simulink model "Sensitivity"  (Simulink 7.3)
settings: Solver=ode5  StartTime=0.0  StopTime=100  FixedStep=0.04  RelTol=1e-3
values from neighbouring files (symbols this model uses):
  Ts = 0.04    [run.m]    (also in z2s_transf.m)
undefined symbols (not defined in the file or in its folder): Alfc, Apfc, Azpl, Blfc, Bpfc, Bzpl, Clfc, Cpfc, Czpl, Dlfc, Dpfc, Dzpl, TVC

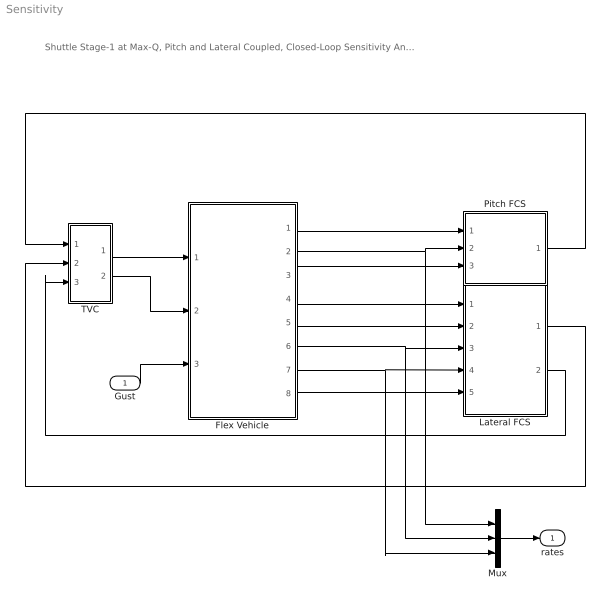
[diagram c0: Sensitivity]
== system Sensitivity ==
  note: Shuttle Stage-1 at Max-Q, Pitch and Lateral Coupled, Closed-Loop Sensitivity Analysis Model
  Gust : Inport  OutDataType=sfix(16)  OutScaling=2^0
  Flex Vehicle : Subsystem
  Lateral FCS : Subsystem
  Mux : Mux  Inputs=3
  Pitch FCS : Subsystem
  TVC : Subsystem
  rates : Outport  OutDataType=sfix(16)  OutScaling=2^0
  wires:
  Pitch FCS/1(DQ_TVC) -> TVC/1(ptch)
  Lateral FCS/1(DP_TVC) -> TVC/2(roll)
  Lateral FCS/2(DR_TVC) -> TVC/3(yaw)
  TVC/2(dz) -> Flex Vehicle/2(dzc)
  TVC/1(dy) -> Flex Vehicle/1(dyc)
  Flex Vehicle/2(q-flx) -> Mux/1, Pitch FCS/2(q)
  Flex Vehicle/3(Nz) -> Pitch FCS/3(Nz)
  Flex Vehicle/4(phi) -> Lateral FCS/1(phi-er)
  Flex Vehicle/5(psi) -> Lateral FCS/2(psi-er)
  Flex Vehicle/6(p-flx) -> Mux/2, Lateral FCS/3(p)
  Flex Vehicle/7(r-flx) -> Mux/3, Lateral FCS/4(r)
  Flex Vehicle/8(Ny) -> Lateral FCS/5(Ny)
  Gust/1 -> Flex Vehicle/3(WG)
  Mux/1 -> rates/1
  Flex Vehicle/1(theta) -> Pitch FCS/1(theta)

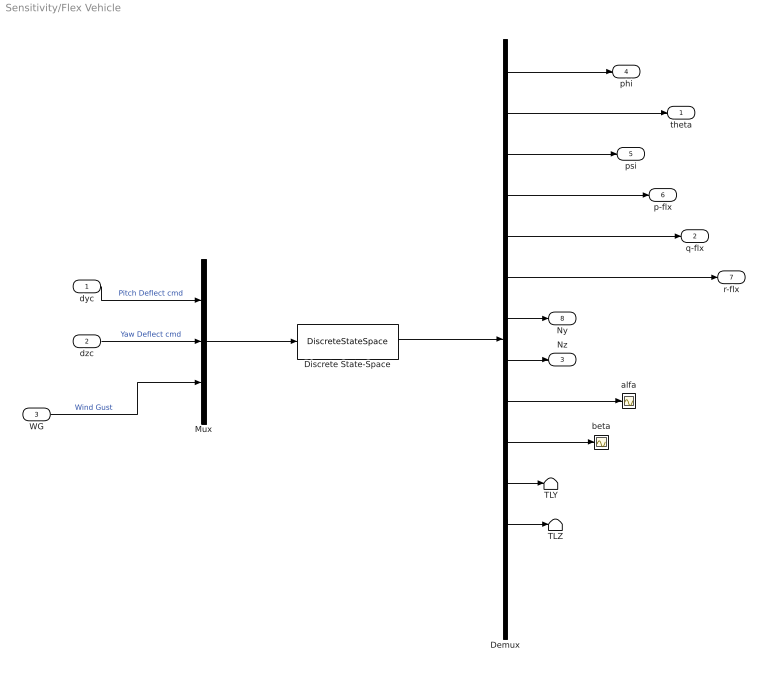
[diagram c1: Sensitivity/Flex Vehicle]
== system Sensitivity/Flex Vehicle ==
  dyc : Inport  PortDimensions=5  OutDataType=sfix(16)  OutScaling=2^0
  dzc : Inport  Port=2  PortDimensions=5  OutDataType=sfix(16)  OutScaling=2^0
  WG : Inport  Port=3  OutDataType=sfix(16)  OutScaling=2^0
  Demux : Demux  Outputs=[1,1,1,1,1,1,1,1,1,1, 5,5,5,5]
  Discrete State-Space : DiscreteStateSpace  A=Azpl  B=Bzpl  C=Czpl  D=Dzpl  SampleTime=Ts
  Mux : Mux  Inputs="[5  5  1]"
  TLY : Terminator
  TLZ : Terminator
  alfa : Scope
  beta : Scope
  theta : Outport  OutDataType=sfix(16)  OutScaling=2^0
  q-flx : Outport  Port=2  OutDataType=sfix(16)  OutScaling=2^0
  Nz : Outport  Port=3  OutDataType=sfix(16)  OutScaling=2^0
  phi : Outport  Port=4  OutDataType=sfix(16)  OutScaling=2^0
  psi : Outport  Port=5  OutDataType=sfix(16)  OutScaling=2^0
  p-flx : Outport  Port=6  OutDataType=sfix(16)  OutScaling=2^0
  r-flx : Outport  Port=7  OutDataType=sfix(16)  OutScaling=2^0
  Ny : Outport  Port=8  OutDataType=sfix(16)  OutScaling=2^0
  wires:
  dyc/1 -> Mux/1  "Pitch Deflect cmd"
  dzc/1 -> Mux/2  "Yaw Deflect cmd"
  WG/1 -> Mux/3  "Wind Gust"
  Mux/1 -> Discrete State-Space/1
  Discrete State-Space/1 -> Demux/1
  Demux/1 -> phi/1
  Demux/2 -> theta/1
  Demux/3 -> psi/1
  Demux/4 -> p-flx/1
  Demux/5 -> q-flx/1
  Demux/6 -> r-flx/1
  Demux/7 -> Ny/1
  Demux/8 -> Nz/1
  Demux/9 -> alfa/1
  Demux/10 -> beta/1
  Demux/11 -> TLY/1
  Demux/12 -> TLZ/1

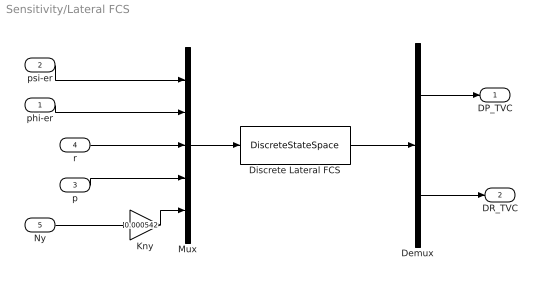
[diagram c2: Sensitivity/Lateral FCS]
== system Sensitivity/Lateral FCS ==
  phi-er : Inport  OutDataType=sfix(16)  OutScaling=2^0
  psi-er : Inport  Port=2  OutDataType=sfix(16)  OutScaling=2^0
  p : Inport  Port=3  OutDataType=sfix(16)  OutScaling=2^0
  r : Inport  Port=4  OutDataType=sfix(16)  OutScaling=2^0
  Ny : Inport  Port=5  OutDataType=sfix(16)  OutScaling=2^0
  Demux : Demux  Outputs=2
  Discrete Lateral FCS : DiscreteStateSpace  A=Alfc  B=Blfc  C=Clfc  D=Dlfc  SampleTime=Ts
  Kny : Gain  Gain=0.000542  ParameterDataType=sfix(16)  ParameterScaling=2^0  OutDataType=sfix(16)  OutScaling=2^0
  Mux : Mux  Inputs=5
  DP_TVC : Outport  OutDataType=sfix(16)  OutScaling=2^0
  DR_TVC : Outport  Port=2  OutDataType=sfix(16)  OutScaling=2^0
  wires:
  psi-er/1 -> Mux/1
  phi-er/1 -> Mux/2
  r/1 -> Mux/3
  Mux/1 -> Discrete Lateral FCS/1
  Discrete Lateral FCS/1 -> Demux/1
  Demux/1 -> DP_TVC/1
  Demux/2 -> DR_TVC/1
  p/1 -> Mux/4
  Ny/1 -> Kny/1
  Kny/1 -> Mux/5

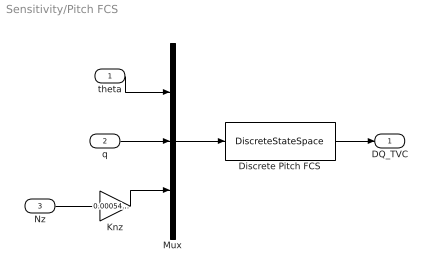
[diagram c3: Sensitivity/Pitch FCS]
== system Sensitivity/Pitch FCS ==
  theta : Inport  OutDataType=sfix(16)  OutScaling=2^0
  q : Inport  Port=2  OutDataType=sfix(16)  OutScaling=2^0
  Nz : Inport  Port=3  OutDataType=sfix(16)  OutScaling=2^0
  Discrete Pitch FCS : DiscreteStateSpace  A=Apfc  B=Bpfc  C=Cpfc  D=Dpfc  SampleTime=Ts
  Knz : Gain  Gain=0.000542*0.5  ParameterDataType=sfix(16)  ParameterScaling=2^0  OutDataType=sfix(16)  OutScaling=2^0
  Mux : Mux  Inputs=3
  DQ_TVC : Outport  OutDataType=sfix(16)  OutScaling=2^0
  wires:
  Mux/1 -> Discrete Pitch FCS/1
  Nz/1 -> Knz/1
  q/1 -> Mux/2
  theta/1 -> Mux/1
  Discrete Pitch FCS/1 -> DQ_TVC/1
  Knz/1 -> Mux/3

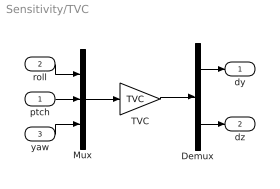
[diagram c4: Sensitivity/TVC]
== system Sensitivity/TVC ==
  ptch : Inport  OutDataType=sfix(16)  OutScaling=2^0
  roll : Inport  Port=2  OutDataType=sfix(16)  OutScaling=2^0
  yaw : Inport  Port=3  OutDataType=sfix(16)  OutScaling=2^0
  Demux : Demux  Outputs="[5  5]"
  Mux : Mux  Inputs=3
  TVC : Gain  Gain=TVC  Multiplication=Matrix(K*u) (u vector)  ParameterDataType=sfix(16)  ParameterScaling=2^0  OutDataType=sfix(16)  OutScaling=2^0
  dy : Outport  OutDataType=sfix(16)  OutScaling=2^0
  dz : Outport  Port=2  OutDataType=sfix(16)  OutScaling=2^0
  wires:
  TVC/1 -> Demux/1
  Mux/1 -> TVC/1
  roll/1 -> Mux/1
  Demux/1 -> dy/1
  ptch/1 -> Mux/2
  Demux/2 -> dz/1
  yaw/1 -> Mux/3
